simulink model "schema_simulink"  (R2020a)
settings: Solver=VariableStepAuto  StartTime=0.0  StopTime=3  RelTol=1e-3
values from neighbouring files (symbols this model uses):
  K = 6050    [script_matlab.m]
  T = 0.0040    (= 0.004)    [script_matlab.m]
undefined symbols (not defined in the file or in its folder): denGs, denRs, denRz, numGs, numRs, numRz

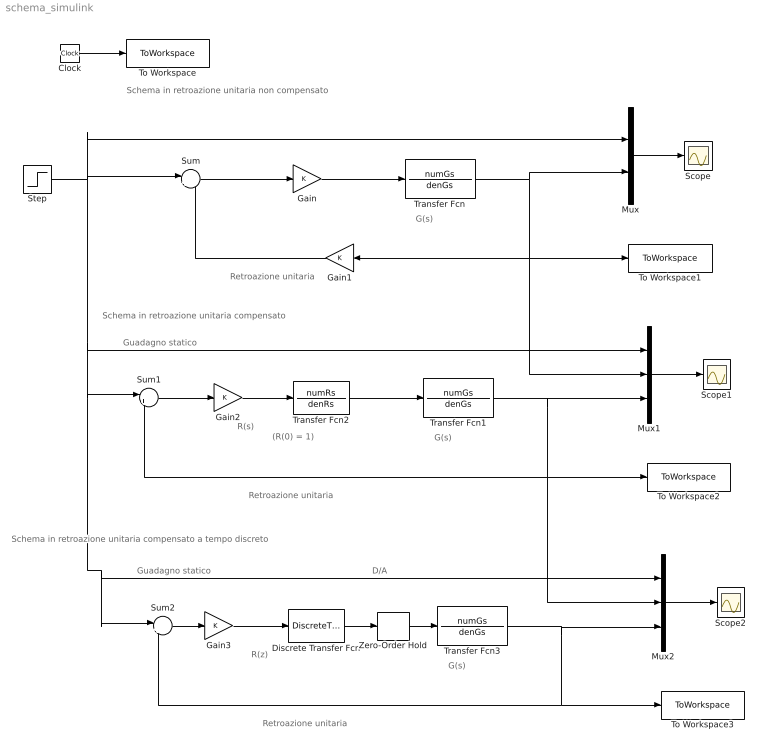
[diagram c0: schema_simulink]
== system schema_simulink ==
  note: D/A
  note: Guadagno statico
  note: (R(0) = 1)
  note: R(s)
  note: Retroazione unitaria
  note: Schema in retroazione unitaria non compensato
  note: G(s)
  note: Retroazione unitaria
  note: Schema in retroazione unitaria compensato
  note: G(s)
  note: Retroazione unitaria
  note: Schema in retroazione unitaria compensato a tempo discreto
  note: Guadagno statico
  note: R(z)
  note: G(s)
  Clock : Clock
  Discrete Transfer Fcn : DiscreteTransferFcn  Numerator=numRz  Denominator=denRz  SampleTime=T
  Gain : Gain
  Gain1 : Gain
  Gain2 : Gain  Gain=K
  Gain3 : Gain  Gain=K
  Mux : Mux  Inputs=2
  Mux1 : Mux  Inputs=3
  Mux2 : Mux  Inputs=3
  Scope : Scope
  Scope1 : Scope
  Scope2 : Scope
  Step : Step  Time=0  SampleTime=0
  Sum : Sum  Inputs=|+-
  Sum1 : Sum  Inputs=|+-
  Sum2 : Sum  Inputs=|+-
  To Workspace : ToWorkspace  VariableName=tsim  SampleTime=-1
  To Workspace1 : ToWorkspace  VariableName=ync  SampleTime=-1
  To Workspace2 : ToWorkspace  VariableName=yc  SampleTime=-1
  To Workspace3 : ToWorkspace  VariableName=yd  SampleTime=-1
  Transfer Fcn : TransferFcn  Numerator=numGs  Denominator=denGs
  Transfer Fcn1 : TransferFcn  Numerator=numGs  Denominator=denGs
  Transfer Fcn2 : TransferFcn  Numerator=numRs  Denominator=denRs
  Transfer Fcn3 : TransferFcn  Numerator=numGs  Denominator=denGs
  Zero-Order Hold : ZeroOrderHold  SampleTime=T
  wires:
  Transfer Fcn/1 -> Mux/2, To Workspace1/1, Mux1/2, Gain1/1
  Mux/1 -> Scope/1
  Clock/1 -> To Workspace/1
  Sum/1 -> Gain/1
  Gain/1 -> Transfer Fcn/1
  Gain1/1 -> Sum/2
  Mux1/1 -> Scope1/1
  Transfer Fcn2/1 -> Transfer Fcn1/1
  Sum1/1 -> Gain2/1
  Gain2/1 -> Transfer Fcn2/1
  Zero-Order Hold/1 -> Transfer Fcn3/1
  Transfer Fcn3/1 -> Mux2/3, Sum2/2, To Workspace3/1
  Mux2/1 -> Scope2/1
  Gain3/1 -> Discrete Transfer Fcn/1
  Sum2/1 -> Gain3/1
  Transfer Fcn1/1 -> Mux1/3, Mux2/2, Sum1/2, To Workspace2/1
  Step/1 -> Sum/1, Sum2/1, Mux2/1, Sum1/1, Mux1/1, Mux/1
  Discrete Transfer Fcn/1 -> Zero-Order Hold/1
